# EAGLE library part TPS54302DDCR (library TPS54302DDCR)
Conv DC-DC 4.5V to 28V Synchronous Step Down Single-Out 0.6V to 26V 3A 6-Pin TSOT-23 T/R Source: Datasheet
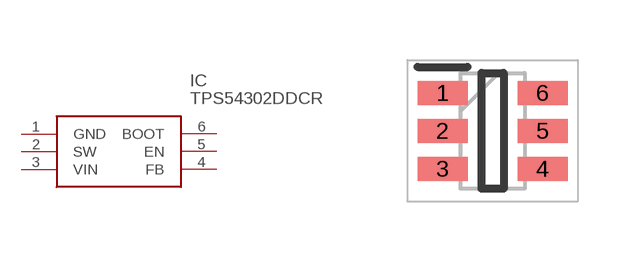
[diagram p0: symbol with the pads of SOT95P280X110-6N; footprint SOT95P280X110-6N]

Designator prefix IC

## TPS54302DDCR (Description: Conv DC-DC 4.5V to 28V Synchronous Step Down Single-Out 0.6V to 26V 3A 6-Pin TSOT-23 T/R; Height: 1.1mm; Manufacturer_Name: Texas Instruments; Manufacturer_Part_Number: TPS54302DDCR; Mouser_Part_Number: 595-TPS54302DDCR; Mouser_Price-Stock: https://www.mouser.co.uk/ProductDetail/Texas-Instruments/TPS54302DDCR?qs=zEmsApcVOkUXM7UP0GSO2g%3D%3D)  [SOT95P280X110-6N]
1  GND
2  SW
3  VIN
4  FB
5  EN
6  BOOT

## Footprint SOT95P280X110-6N (pad centres in mm)
DDC
smd 1.25 x 0.6: 1 -1.25,0.95; 2 -1.25,0; 3 -1.25,-0.95; 4 1.25,-0.95; 5 1.25,0; 6 1.25,0.95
